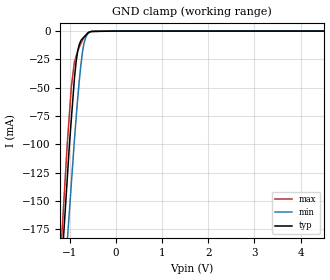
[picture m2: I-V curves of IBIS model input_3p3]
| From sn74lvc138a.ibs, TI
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|   input_3p3 Model
[Model]   input_3p3
Model_type   Input
Vinl = 0.8
Vinh = 2.0
|   typ   min   max
|   (nom PVT)   (fast PVT)   (slow PVT)
|C_comp from frequency sweep method (F=10MHz)
|Average
|C_comp   3.258e-12   3.243e-12   3.428e-12
|C_comp from LC tank measurement(L=1nH)
|Average
|Resonant Frequency(Hz)   3.110e+09   3.120e+09   3.110e+09
C_comp   2.622e-12   2.605e-12   2.622e-12
| Where nom  PVT is Nominal Process, 3.3V, 27C
|   Fast PVT is Strong Process,  3.6V, -40C
|   Slow PVT is Weak Process,   3V, 125C
[Voltage Range]   3.3   3   3.6
|Ambient Temperature   25   85   -40
|Junction Temperature
[Temperature Range]   27   125   -40
[Power Clamp Reference]   3.3   3   3.6
[GND Clamp Reference]   0   0   0
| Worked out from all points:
|   GND clamp passes 1 mA (typ) near -0.59 V on its own axis
[GND Clamp]
|   Voltage   I(typ)   I(min)   I(max)
-3.3V     -1.79A     -1.738A    -1.84A
-1.206V   -230.5mA   -281.9mA   -205mA
-1.158V   -197.7mA   -251.7mA   -172.2mA
-1.058V   -133.9mA   -190mA     -103.5mA
-1.035V   -119mA     -175.6mA   -89.77mA
-964.8mV  -78.06mA   -135.1mA   -49.43mA
-897.6mV  -41.85mA   -96.26mA   -27.47mA
-828.3mV  -17.98mA   -60.45mA   -18.05mA
-717mV    -6.418mA   -16.93mA   -7.441mA
-657mV    -3.886mA   -5.856mA   -3.906mA
-590.7mV  -1.089mA   -1.655mA   -1.329mA
6.6V      0A         0A         0A
[POWER Clamp]
|   Voltage   I(typ)   I(min)   I(max)
-3.3V     0A         0A         0A
0V        0A         0A         0A
6.6V      0A         0A         0A
